| This Model is valid for Automotive grade 2 Temperature Range -40C<=Tc<=105C
| Valid for LPDDR4-4266 operation
| Part Number   VDD/VDDQ   Package   Architecture
| SCB11N8G322BF-04ZA2   1.1 +0.07/-0.04  BGA   8G bit x 32
[IBIS ver] 5.0
[File name]  usssn8g32ba2.ibs
[File Rev]  1.0
[Date]   October 8, 2023
[Source] Simulation of a silicon level SPICE model
[Notes]  IBIS Characteristics for I/O Buffer
  IBIS Model Revision History: Rev 1.0:
  2023-10-08 - IBIS model file initial creation
[Disclaimer]  The IBIS models are for modeling purpose only and are subject to change without any notice. UniIC is not
  responsible for any problems the models may cause.
[Copyright] Copyright 2023 UniIC Semiconductors Corp. All rights reserved
|   Component SCB11N8G322BF-04ZA2
[Component] SCB11N8G322BF-04ZA2
[Manufacturer] UniIC Semiconductors Corp.
[Package]
| variable   typ   min   max
R_pkg   0.750   0.698   0.832
L_pkg   1.500nH   1.330nH   1.720nH
C_pkg   0.630pF   0.579pF   0.668pF
[Pin]  signal_name   model_name   R_pin   L_pin   C_pin
A1   DNU   NC
A2   DNU   NC
A3   VSS   Gnd
A4   VDD2   Power
A5   ZQ0   NC
A8   DNU   NC
A9   VDD2   Power
A10   VSS   Gnd
A11   DNU   NC
A12   DNU   NC
AA1   DNU   NC
AA2   DQ0_B   DQ   0.835   1.840nH   0.572pF
AA3   VDDQ   Power
AA4   DQ7_B   DQ   0.804   1.770nH   0.584pF
AA5   VDDQ   Power
AA8   VDDQ   Power
AA9   DQ15_B   DQ   0.820   1.780nH   0.582pF
AA10   VDDQ   Power
AA11   DQ8_B   DQ   0.835   1.830nH   0.564pF
AA12   DNU   NC
AB1   DNU   NC
AB2   DNU   NC
AB3   VSS   Gnd
AB4   VDD2   Power
AB5   VSS   Gnd
AB8   VSS   Gnd
AB9   VDD2   Power
AB10   VSS   Gnd
AB11   DNU   NC
AB12   DNU   NC
B1   DNU   NC
B2   DQ0_A   DQ   0.825   1.680nH   0.658pF
B3   VDDQ   Power
B4   DQ7_A   DQ   0.810   1.640nH   0.579pF
B5   VDDQ   Power
B8   VDDQ   Power
B9   DQ15_A   DQ   0.819   1.720nH   0.645pF
B10   VDDQ   Power
B11   DQ8_A   DQ   0.832   1.650nH   0.595pF
B12   DNU   NC
C1   VSS   Gnd
C2   DQ1_A   DQ   0.809   1.620nH   0.658pF
C3   DMI0_A   DQ   0.816   1.600nH   0.644pF
C4   DQ6_A   DQ   0.782   1.720nH   0.645pF
C5   VSS   Gnd
C8   VSS   Gnd
C9   DQ14_A   DQ   0.776   1.550nH   0.639pF
C10   DMI1_A   DQ   0.793   1.560nH   0.644pF
C11   DQ9_A   DQ   0.809   1.640nH   0.668pF
C12   VSS   Gnd
D1   VDDQ   Power
D2   VSS   Gnd
D3   DQS0_T_A   DQS   0.752   1.480nH   0.614pF
D4   VSS   Gnd
D5   VDDQ   Power
D8   VDDQ   Power
D9   VSS   Gnd
D10   DQS1_T_A   DQS   0.750   1.460nH   0.630pF
D11   VSS   Gnd
D12   VDDQ   Power
E1   VSS   Gnd
E2   DQ2_A   DQ   0.772   1.490nH   0.579pF
E3   DQS0_C_A   DQS   0.739   1.480nH   0.613pF
E4   DQ5_A   DQ   0.698   1.360nH   0.629pF
E5   VSS   Gnd
E8   VSS   Gnd
E9   DQ13_A   DQ   0.701   1.330nH   0.647pF
E10   DQS1_C_A   DQS   0.749   1.470nH   0.622pF
E11   DQ10_A   DQ   0.786   1.530nH   0.591pF
E12   VSS   Gnd
F1   VDD1   Power
F2   DQ3_A   DQ   0.748   1.480nH   0.582pF
F3   VDDQ   Power
F4   DQ4_A   DQ   0.740   1.430nH   0.640pF
F5   VDD2   Power
F8   VDD2   Power
F9   DQ12_A   DQ   0.751   1.420nH   0.664pF
F10   VDDQ   Power
F11   DQ11_A   DQ   0.765   1.520nH   0.562pF
F12   VDD1   Power
G1   VSS   Gnd
G2   ODTCA_A   RCV_RST_N
G3   VSS   Gnd
G4   VDD1   Power
G5   VSS   Gnd
G8   VSS   Gnd
G9   VDD1   Power
G10   VSS   Gnd
G11   ZQ2   NC
G12   VSS   Gnd
H1   VDD2   Power
H2   CA0_A   CA   1.640   2.810nH   1.140pF
H3   DNU   NC
H4   CS0_A   CA   1.170   2.210nH   0.905pF
H5   VDD2   Power
H8   VDD2   Power
H9   CA2_A   CA   1.550   2.690nH   1.150pF
H10   CA3_A   CA   1.570   2.740nH   1.120pF
H11   CA4_A   CA   1.600   2.780nH   1.160pF
H12   VDD2   Power
J1   VSS   Gnd
J2   CA1_A   CA   1.670   2.970nH   1.170pF
J3   VSS   Gnd
J4   CKE0_A   RCV_CKE   1.490   2.670nH   1.000pF
J5   DNU   NC
J8   CKT_A   CLK   1.400   2.570nH   1.060pF
J9   CKC_A   CLK   1.420   2.610nH   1.070pF
J10   VSS   Gnd
J11   CA5_A   CA   1.710   2.940nH   1.200pF
J12   VSS   Gnd
K1   VDD2   Power
K2   VSS   Gnd
K3   VDD2   Power
K4   VSS   Gnd
K5   DNU   NC
K8   DNU   NC
K9   VSS   Gnd
K10   VDD2   Power
K11   VSS   Gnd
K12   VDD2   Power
N1   VDD2   Power
N2   VSS   Gnd
N3   VDD2   Power
N4   VSS   Gnd
N5   DNU   NC
N8   DNU   NC
N9   VSS   Gnd
N10   VDD2   Power
N11   VSS   Gnd
N12   VDD2   Power
P1   VSS   Gnd
P2   CA1_B   CA   1.640   4.130nH   1.160pF
P3   VSS   Gnd
P4   CKE0_B   RCV_CKE   1.370   3.590nH   1.000pF
P5   DNU   NC
P8   CKT_B   CLK   1.360   3.150nH   1.070pF
P9   CKC_B   CLK   1.420   3.190nH   1.070pF
P10   VSS   Gnd
P11   CA5_B   CA   1.610   3.550nH   1.170pF
P12   VSS   Gnd
R1   VDD2   Power
R2   CA0_B   CA   1.570   3.920nH   1.110pF
R3   NC   NC
R4   CS0_B   CA   1.240   3.090nH   0.917pF
R5   VDD2   Power
R8   VDD2   Power
R9   CA2_B   CA   1.560   3.330nH   1.170pF
R10   CA3_B   CA   1.520   3.350nH   1.140pF
R11   CA4_B   CA   1.660   3.620nH   1.200pF
R12   VDD2   Power
T1   VSS   Gnd
T2   ODTCA_B   RCV_RST_N
T3   VSS   Gnd
T4   VDD1   Power
T5   VSS   Gnd
T8   VSS   Gnd
T9   VDD1   Power
T10   VSS   Gnd
T11   RESET_N   RCV_RST_N
T12   VSS   Gnd
U1   VDD1   Power
U2   DQ3_B   DQ   0.792   1.670nH   0.563pF
U3   VDDQ   Power
U4   DQ4_B   DQ   0.775   1.610nH   0.550pF
U5   VDD2   Power
U8   VDD2   Power
U9   DQ12_B   DQ   0.731   1.520nH   0.585pF
U10   VDDQ   Power
U11   DQ11_B   DQ   0.795   1.670nH   0.572pF
U12   VDD1   Power
V1   VSS   Gnd
V2   DQ2_B   DQ   0.790   1.640nH   0.565pF
V3   DQS0_C_B   DQS   0.777   1.590nH   0.612pF
V4   DQ5_B   DQ   0.750   1.510nH   0.652pF
V5   VSS   Gnd
V8   VSS   Gnd
V9   DQ13_B   DQ   0.724   1.500nH   0.648pF
V10   DQS1_C_B   DQS   0.772   1.610nH   0.610pF
V11   DQ10_B   DQ   0.834   1.690nH   0.610pF
V12   VSS   Gnd
W1   VDDQ   Power
W2   VSS   Gnd
W3   DQS0_T_B   DQS   0.780   1.610nH   0.610pF
W4   VSS   Gnd
W5   VDDQ   Power
W8   VDDQ   Power
W9   VSS   Gnd
W10   DQS1_T_B   DQS   0.767   1.590nH   0.614pF
W11   VSS   Gnd
W12   VDDQ   Power
Y1   VSS   Gnd
Y2   DQ1_B   DQ   0.822   1.760nH   0.644pF
Y3   DMI0_B   DQ   0.812   1.630nH   0.623pF
Y4   DQ6_B   DQ   0.807   1.700nH   0.631pF
Y5   VSS   Gnd
Y8   VSS   Gnd
Y9   DQ14_B   DQ   0.841   1.720nH   0.647pF
Y10   DMI1_B   DQ   0.781   1.630nH   0.623pF
Y11   DQ9_B   DQ   0.834   1.770nH   0.633pF
Y12   VSS   Gnd
|IN   dq_in   dummy
|EN   dq_en   dummy
[Diff pin]  inv_pin  vdiff   tdelay_typ   tdelay_min   tdelay_max
D3   E3   0.160V   NA   NA   NA
D10   E10   0.160V   NA   NA   NA
J8   J9   0.160V   NA   NA   NA
V3   W3   0.160V   NA   NA   NA
V10   W10   0.160V   NA   NA   NA
P8   P9   0.160V   NA   NA   NA
[Model Selector] DQ
DQ_PU_PD_480_240_DRIVE_SOCODT240_VOH33  voh=vddq/3, 480 Ohm Pullup, 240 Ohm Pulldown,240ohm SOCODT
DQ_PU_PD_480_120_DRIVE_SOCODT240_VOH33  voh=vddq/3, 480 Ohm Pullup, 120 Ohm Pulldown,240ohm SOCODT
DQ_PU_PD_480_80_DRIVE_SOCODT240_VOH33  voh=vddq/3, 480 Ohm Pullup, 80 Ohm Pulldown,240ohm SOCODT
DQ_PU_PD_480_60_DRIVE_SOCODT240_VOH33  voh=vddq/3, 480 Ohm Pullup, 60 Ohm Pulldown,240ohm SOCODT
DQ_PU_PD_480_48_DRIVE_SOCODT240_VOH33  voh=vddq/3, 480 Ohm Pullup, 48 Ohm Pulldown,240ohm SOCODT
DQ_PU_PD_480_40_DRIVE_SOCODT240_VOH33  voh=vddq/3, 480 Ohm Pullup, 40 Ohm Pulldown,240ohm SOCODT
DQ_PU_PD_240_240_DRIVE_SOCODT120_VOH33  voh=vddq/3, 240 Ohm Pullup, 240 Ohm Pulldown,120ohm SOCODT
DQ_PU_PD_240_120_DRIVE_SOCODT120_VOH33  voh=vddq/3, 240 Ohm Pullup, 120 Ohm Pulldown,120ohm SOCODT
DQ_PU_PD_240_80_DRIVE_SOCODT120_VOH33  voh=vddq/3, 240 Ohm Pullup, 80 Ohm Pulldown,120ohm SOCODT
DQ_PU_PD_240_60_DRIVE_SOCODT120_VOH33  voh=vddq/3, 240 Ohm Pullup, 60 Ohm Pulldown,120ohm SOCODT
DQ_PU_PD_240_48_DRIVE_SOCODT120_VOH33  voh=vddq/3, 240 Ohm Pullup, 48 Ohm Pulldown,120ohm SOCODT
DQ_PU_PD_240_40_DRIVE_SOCODT120_VOH33  voh=vddq/3, 240 Ohm Pullup, 40 Ohm Pulldown,120ohm SOCODT
DQ_PU_PD_160_240_DRIVE_SOCODT80_VOH33  voh=vddq/3, 160 Ohm Pullup, 240 Ohm Pulldown,80ohm SOCODT
DQ_PU_PD_160_120_DRIVE_SOCODT80_VOH33  voh=vddq/3, 160 Ohm Pullup, 120 Ohm Pulldown,80ohm SOCODT
DQ_PU_PD_160_80_DRIVE_SOCODT80_VOH33  voh=vddq/3, 160 Ohm Pullup, 80 Ohm Pulldown,80ohm SOCODT
DQ_PU_PD_160_60_DRIVE_SOCODT80_VOH33  voh=vddq/3, 160 Ohm Pullup, 60 Ohm Pulldown,80ohm SOCODT
DQ_PU_PD_160_48_DRIVE_SOCODT80_VOH33  voh=vddq/3, 160 Ohm Pullup, 48 Ohm Pulldown,80ohm SOCODT
DQ_PU_PD_160_40_DRIVE_SOCODT80_VOH33  voh=vddq/3, 160 Ohm Pullup, 40 Ohm Pulldown,80ohm SOCODT
DQ_PU_PD_120_240_DRIVE_SOCODT60_VOH33  voh=vddq/3, 120 Ohm Pullup, 240 Ohm Pulldown,60ohm SOCODT
DQ_PU_PD_120_120_DRIVE_SOCODT60_VOH33  voh=vddq/3, 120 Ohm Pullup, 120 Ohm Pulldown,60ohm SOCODT
DQ_PU_PD_120_80_DRIVE_SOCODT60_VOH33  voh=vddq/3, 120 Ohm Pullup, 80 Ohm Pulldown,60ohm SOCODT
DQ_PU_PD_120_60_DRIVE_SOCODT60_VOH33  voh=vddq/3, 120 Ohm Pullup, 60 Ohm Pulldown,60ohm SOCODT
DQ_PU_PD_120_48_DRIVE_SOCODT60_VOH33  voh=vddq/3, 120 Ohm Pullup, 48 Ohm Pulldown,60ohm SOCODT
DQ_PU_PD_120_40_DRIVE_SOCODT60_VOH33  voh=vddq/3, 120 Ohm Pullup, 40 Ohm Pulldown,60ohm SOCODT
DQ_PU_PD_96_240_DRIVE_SOCODT48_VOH33  voh=vddq/3, 96 Ohm Pullup, 240 Ohm Pulldown,48ohm SOCODT
DQ_PU_PD_96_120_DRIVE_SOCODT48_VOH33  voh=vddq/3, 96 Ohm Pullup, 120 Ohm Pulldown,48ohm SOCODT
DQ_PU_PD_96_80_DRIVE_SOCODT48_VOH33  voh=vddq/3, 96 Ohm Pullup, 80 Ohm Pulldown,48ohm SOCODT
DQ_PU_PD_96_60_DRIVE_SOCODT48_VOH33  voh=vddq/3, 96 Ohm Pullup, 60 Ohm Pulldown,48ohm SOCODT
DQ_PU_PD_96_48_DRIVE_SOCODT48_VOH33  voh=vddq/3, 96 Ohm Pullup, 48 Ohm Pulldown,48ohm SOCODT
DQ_PU_PD_96_40_DRIVE_SOCODT48_VOH33  voh=vddq/3, 96 Ohm Pullup, 40 Ohm Pulldown,48ohm SOCODT
DQ_PU_PD_80_240_DRIVE_SOCODT40_VOH33  voh=vddq/3, 80 Ohm Pullup, 240 Ohm Pulldown,SOCODT disable OR 40ohm SOCODT
DQ_PU_PD_80_120_DRIVE_SOCODT40_VOH33  voh=vddq/3, 80 Ohm Pullup, 120 Ohm Pulldown,SOCODT disable OR 40ohm SOCODT
DQ_PU_PD_80_80_DRIVE_SOCODT40_VOH33  voh=vddq/3, 80 Ohm Pullup, 80 Ohm Pulldown,SOCODT disable OR 40ohm SOCODT
DQ_PU_PD_80_60_DRIVE_SOCODT40_VOH33  voh=vddq/3, 80 Ohm Pullup, 60 Ohm Pulldown,SOCODT disable OR 40ohm SOCODT
DQ_PU_PD_80_48_DRIVE_SOCODT40_VOH33  voh=vddq/3, 80 Ohm Pullup, 48 Ohm Pulldown,SOCODT disable OR 40ohm SOCODT
DQ_PU_PD_80_40_DRIVE_SOCODT40_VOH33  voh=vddq/3, 80 Ohm Pullup, 40 Ohm Pulldown,SOCODT disable OR 40ohm SOCODT
DQ_PU_PD_120_240_DRIVE_SOCODT80_VOH40  voh=vddq/2.5, 120 Ohm Pullup, 240 Ohm Pulldown,SOCODT disable OR 80ohm SOCODT
DQ_PU_PD_120_120_DRIVE_SOCODT80_VOH40  voh=vddq/2.5, 120 Ohm Pullup, 120 Ohm Pulldown,SOCODT disable OR 80ohm SOCODT
DQ_PU_PD_120_80_DRIVE_SOCODT80_VOH40  voh=vddq/2.5, 120 Ohm Pullup, 80 Ohm Pulldown,SOCODT disable OR 80ohm SOCODT
DQ_PU_PD_120_60_DRIVE_SOCODT80_VOH40  voh=vddq/2.5, 120 Ohm Pullup, 60 Ohm Pulldown,SOCODT disable OR 80ohm SOCODT
DQ_PU_PD_120_48_DRIVE_SOCODT80_VOH40  voh=vddq/2.5, 120 Ohm Pullup, 48 Ohm Pulldown,SOCODT disable OR 80ohm SOCODT
DQ_PU_PD_120_40_DRIVE_SOCODT80_VOH40  voh=vddq/2.5, 120 Ohm Pullup, 40 Ohm Pulldown,SOCODT disable OR 80ohm SOCODT
DQ_PU_PD_180_240_DRIVE_SOCODT120_VOH40  voh=vddq/2.5, 180 Ohm Pullup, 240 Ohm Pulldown,120ohm SOCODT
DQ_PU_PD_180_120_DRIVE_SOCODT120_VOH40  voh=vddq/2.5, 180 Ohm Pullup, 120 Ohm Pulldown,120ohm SOCODT
DQ_PU_PD_180_80_DRIVE_SOCODT120_VOH40  voh=vddq/2.5, 180 Ohm Pullup, 80 Ohm Pulldown,120ohm SOCODT
DQ_PU_PD_180_60_DRIVE_SOCODT120_VOH40  voh=vddq/2.5, 180 Ohm Pullup, 60 Ohm Pulldown,120ohm SOCODT
DQ_PU_PD_180_48_DRIVE_SOCODT120_VOH40  voh=vddq/2.5, 180 Ohm Pullup, 48 Ohm Pulldown,120ohm SOCODT
DQ_PU_PD_180_40_DRIVE_SOCODT120_VOH40  voh=vddq/2.5, 180 Ohm Pullup, 40 Ohm Pulldown,120ohm SOCODT
DQ_PU_PD_360_240_DRIVE_SOCODT240_VOH40  voh=vddq/2.5, 360 Ohm Pullup, 240 Ohm Pulldown,240ohm SOCODT
DQ_PU_PD_360_120_DRIVE_SOCODT240_VOH40  voh=vddq/2.5, 360 Ohm Pullup, 120 Ohm Pulldown,240ohm SOCODT
DQ_PU_PD_360_80_DRIVE_SOCODT240_VOH40  voh=vddq/2.5, 360 Ohm Pullup, 80 Ohm Pulldown,240ohm SOCODT
DQ_PU_PD_360_60_DRIVE_SOCODT240_VOH40  voh=vddq/2.5, 360 Ohm Pullup, 60 Ohm Pulldown,240ohm SOCODT
DQ_PU_PD_360_48_DRIVE_SOCODT240_VOH40  voh=vddq/2.5, 360 Ohm Pullup, 48 Ohm Pulldown,240ohm SOCODT
DQ_PU_PD_360_40_DRIVE_SOCODT240_VOH40  voh=vddq/2.5, 360 Ohm Pullup, 40 Ohm Pulldown,240ohm SOCODT
DQ_ODTOFF  DQ Type input, ODT off for DQ_RCV
DQ_ODT40_VOH33  voh=vddq/3, DQ Type input, ODT 40 for DQ_RCV
DQ_ODT48_VOH33  voh=vddq/3, DQ Type input, ODT 48 for DQ_RCV
DQ_ODT60_VOH33  voh=vddq/3, DQ Type input, ODT 60 for DQ_RCV
DQ_ODT80_VOH33  voh=vddq/3, DQ Type input, ODT 80 for DQ_RCV
DQ_ODT120_VOH33  voh=vddq/3, DQ Type input, ODT 120 for DQ_RCV
DQ_ODT240_VOH33  voh=vddq/3, DQ Type input, ODT 240 for DQ_RCV
DQ_ODT40_VOH40  voh=vddq/2.5, DQ Type input, ODT 40 for DQ_RCV
DQ_ODT48_VOH40  voh=vddq/2.5, DQ Type input, ODT 48 for DQ_RCV
DQ_ODT60_VOH40  voh=vddq/2.5, DQ Type input, ODT 60 for DQ_RCV
DQ_ODT80_VOH40  voh=vddq/2.5, DQ Type input, ODT 80 for DQ_RCV
DQ_ODT120_VOH40  voh=vddq/2.5, DQ Type input, ODT 120 for DQ_RCV
DQ_ODT240_VOH40  voh=vddq/2.5, DQ Type input, ODT 240 for DQ_RCV
[Model Selector] DQS
DQS_PU_PD_480_240_DRIVE_SOCODT240_VOH33  voh=vddq/3, 480 Ohm Pullup, 240 Ohm Pulldown,240ohm SOCODT
DQS_PU_PD_480_120_DRIVE_SOCODT240_VOH33  voh=vddq/3, 480 Ohm Pullup, 120 Ohm Pulldown,240ohm SOCODT
DQS_PU_PD_480_80_DRIVE_SOCODT240_VOH33  voh=vddq/3, 480 Ohm Pullup, 80 Ohm Pulldown,240ohm SOCODT
DQS_PU_PD_480_60_DRIVE_SOCODT240_VOH33  voh=vddq/3, 480 Ohm Pullup, 60 Ohm Pulldown,240ohm SOCODT
DQS_PU_PD_480_48_DRIVE_SOCODT240_VOH33  voh=vddq/3, 480 Ohm Pullup, 48 Ohm Pulldown,240ohm SOCODT
DQS_PU_PD_480_40_DRIVE_SOCODT240_VOH33  voh=vddq/3, 480 Ohm Pullup, 40 Ohm Pulldown,240ohm SOCODT
DQS_PU_PD_240_240_DRIVE_SOCODT120_VOH33  voh=vddq/3, 240 Ohm Pullup, 240 Ohm Pulldown,120ohm SOCODT
DQS_PU_PD_240_120_DRIVE_SOCODT120_VOH33  voh=vddq/3, 240 Ohm Pullup, 120 Ohm Pulldown,120ohm SOCODT
DQS_PU_PD_240_80_DRIVE_SOCODT120_VOH33  voh=vddq/3, 240 Ohm Pullup, 80 Ohm Pulldown,120ohm SOCODT
DQS_PU_PD_240_60_DRIVE_SOCODT120_VOH33  voh=vddq/3, 240 Ohm Pullup, 60 Ohm Pulldown,120ohm SOCODT
DQS_PU_PD_240_48_DRIVE_SOCODT120_VOH33  voh=vddq/3, 240 Ohm Pullup, 48 Ohm Pulldown,120ohm SOCODT
DQS_PU_PD_240_40_DRIVE_SOCODT120_VOH33  voh=vddq/3, 240 Ohm Pullup, 40 Ohm Pulldown,120ohm SOCODT
DQS_PU_PD_160_240_DRIVE_SOCODT80_VOH33  voh=vddq/3, 160 Ohm Pullup, 240 Ohm Pulldown,80ohm SOCODT
DQS_PU_PD_160_120_DRIVE_SOCODT80_VOH33  voh=vddq/3, 160 Ohm Pullup, 120 Ohm Pulldown,80ohm SOCODT
DQS_PU_PD_160_80_DRIVE_SOCODT80_VOH33  voh=vddq/3, 160 Ohm Pullup, 80 Ohm Pulldown,80ohm SOCODT
DQS_PU_PD_160_60_DRIVE_SOCODT80_VOH33  voh=vddq/3, 160 Ohm Pullup, 60 Ohm Pulldown,80ohm SOCODT
DQS_PU_PD_160_48_DRIVE_SOCODT80_VOH33  voh=vddq/3, 160 Ohm Pullup, 48 Ohm Pulldown,80ohm SOCODT
DQS_PU_PD_160_40_DRIVE_SOCODT80_VOH33  voh=vddq/3, 160 Ohm Pullup, 40 Ohm Pulldown,80ohm SOCODT
DQS_PU_PD_120_240_DRIVE_SOCODT60_VOH33  voh=vddq/3, 120 Ohm Pullup, 240 Ohm Pulldown,60ohm SOCODT
DQS_PU_PD_120_120_DRIVE_SOCODT60_VOH33  voh=vddq/3, 120 Ohm Pullup, 120 Ohm Pulldown,60ohm SOCODT
DQS_PU_PD_120_80_DRIVE_SOCODT60_VOH33  voh=vddq/3, 120 Ohm Pullup, 80 Ohm Pulldown,60ohm SOCODT
DQS_PU_PD_120_60_DRIVE_SOCODT60_VOH33  voh=vddq/3, 120 Ohm Pullup, 60 Ohm Pulldown,60ohm SOCODT
DQS_PU_PD_120_48_DRIVE_SOCODT60_VOH33  voh=vddq/3, 120 Ohm Pullup, 48 Ohm Pulldown,60ohm SOCODT
DQS_PU_PD_120_40_DRIVE_SOCODT60_VOH33  voh=vddq/3, 120 Ohm Pullup, 40 Ohm Pulldown,60ohm SOCODT
DQS_PU_PD_96_240_DRIVE_SOCODT48_VOH33  voh=vddq/3, 96 Ohm Pullup, 240 Ohm Pulldown,48ohm SOCODT
DQS_PU_PD_96_120_DRIVE_SOCODT48_VOH33  voh=vddq/3, 96 Ohm Pullup, 120 Ohm Pulldown,48ohm SOCODT
DQS_PU_PD_96_80_DRIVE_SOCODT48_VOH33  voh=vddq/3, 96 Ohm Pullup, 80 Ohm Pulldown,48ohm SOCODT
DQS_PU_PD_96_60_DRIVE_SOCODT48_VOH33  voh=vddq/3, 96 Ohm Pullup, 60 Ohm Pulldown,48ohm SOCODT
DQS_PU_PD_96_48_DRIVE_SOCODT48_VOH33  voh=vddq/3, 96 Ohm Pullup, 48 Ohm Pulldown,48ohm SOCODT
DQS_PU_PD_96_40_DRIVE_SOCODT48_VOH33  voh=vddq/3, 96 Ohm Pullup, 40 Ohm Pulldown,48ohm SOCODT
DQS_PU_PD_80_240_DRIVE_SOCODT40_VOH33  voh=vddq/3, 80 Ohm Pullup, 240 Ohm Pulldown,SOCODT disable OR 40ohm SOCODT
DQS_PU_PD_80_120_DRIVE_SOCODT40_VOH33  voh=vddq/3, 80 Ohm Pullup, 120 Ohm Pulldown,SOCODT disable OR 40ohm SOCODT
DQS_PU_PD_80_80_DRIVE_SOCODT40_VOH33  voh=vddq/3, 80 Ohm Pullup, 80 Ohm Pulldown,SOCODT disable OR 40ohm SOCODT
DQS_PU_PD_80_60_DRIVE_SOCODT40_VOH33  voh=vddq/3, 80 Ohm Pullup, 60 Ohm Pulldown,SOCODT disable OR 40ohm SOCODT
DQS_PU_PD_80_48_DRIVE_SOCODT40_VOH33  voh=vddq/3, 80 Ohm Pullup, 48 Ohm Pulldown,SOCODT disable OR 40ohm SOCODT
DQS_PU_PD_80_40_DRIVE_SOCODT40_VOH33  voh=vddq/3, 80 Ohm Pullup, 40 Ohm Pulldown,SOCODT disable OR 40ohm SOCODT
DQS_PU_PD_120_240_DRIVE_SOCODT80_VOH40  voh=vddq/2.5, 120 Ohm Pullup, 240 Ohm Pulldown,SOCODT disable OR 80ohm SOCODT
DQS_PU_PD_120_120_DRIVE_SOCODT80_VOH40  voh=vddq/2.5, 120 Ohm Pullup, 120 Ohm Pulldown,SOCODT disable OR 80ohm SOCODT
DQS_PU_PD_120_80_DRIVE_SOCODT80_VOH40  voh=vddq/2.5, 120 Ohm Pullup, 80 Ohm Pulldown,SOCODT disable OR 80ohm SOCODT
DQS_PU_PD_120_60_DRIVE_SOCODT80_VOH40  voh=vddq/2.5, 120 Ohm Pullup, 60 Ohm Pulldown,SOCODT disable OR 80ohm SOCODT
DQS_PU_PD_120_48_DRIVE_SOCODT80_VOH40  voh=vddq/2.5, 120 Ohm Pullup, 48 Ohm Pulldown,SOCODT disable OR 80ohm SOCODT
DQS_PU_PD_120_40_DRIVE_SOCODT80_VOH40  voh=vddq/2.5, 120 Ohm Pullup, 40 Ohm Pulldown,SOCODT disable OR 80ohm SOCODT
DQS_PU_PD_180_240_DRIVE_SOCODT120_VOH40  voh=vddq/2.5, 180 Ohm Pullup, 240 Ohm Pulldown,120ohm SOCODT
DQS_PU_PD_180_120_DRIVE_SOCODT120_VOH40  voh=vddq/2.5, 180 Ohm Pullup, 120 Ohm Pulldown,120ohm SOCODT
DQS_PU_PD_180_80_DRIVE_SOCODT120_VOH40  voh=vddq/2.5, 180 Ohm Pullup, 80 Ohm Pulldown,120ohm SOCODT
DQS_PU_PD_180_60_DRIVE_SOCODT120_VOH40  voh=vddq/2.5, 180 Ohm Pullup, 60 Ohm Pulldown,120ohm SOCODT
DQS_PU_PD_180_48_DRIVE_SOCODT120_VOH40  voh=vddq/2.5, 180 Ohm Pullup, 48 Ohm Pulldown,120ohm SOCODT
DQS_PU_PD_180_40_DRIVE_SOCODT120_VOH40  voh=vddq/2.5, 180 Ohm Pullup, 40 Ohm Pulldown,120ohm SOCODT
DQS_PU_PD_360_240_DRIVE_SOCODT240_VOH40  voh=vddq/2.5, 360 Ohm Pullup, 240 Ohm Pulldown,240ohm SOCODT
DQS_PU_PD_360_120_DRIVE_SOCODT240_VOH40  voh=vddq/2.5, 360 Ohm Pullup, 120 Ohm Pulldown,240ohm SOCODT
DQS_PU_PD_360_80_DRIVE_SOCODT240_VOH40  voh=vddq/2.5, 360 Ohm Pullup, 80 Ohm Pulldown,240ohm SOCODT
DQS_PU_PD_360_60_DRIVE_SOCODT240_VOH40  voh=vddq/2.5, 360 Ohm Pullup, 60 Ohm Pulldown,240ohm SOCODT
DQS_PU_PD_360_48_DRIVE_SOCODT240_VOH40  voh=vddq/2.5, 360 Ohm Pullup, 48 Ohm Pulldown,240ohm SOCODT
DQS_PU_PD_360_40_DRIVE_SOCODT240_VOH40  voh=vddq/2.5, 360 Ohm Pullup, 40 Ohm Pulldown,240ohm SOCODT
DQS_ODTOFF  DQS Type input, ODT off for DQS_RCV
DQS_ODT40_VOH33  voh=vddq/3, DQS Type input, ODT 40 for DQS_RCV
DQS_ODT48_VOH33  voh=vddq/3, DQS Type input, ODT 48 for DQS_RCV
DQS_ODT60_VOH33  voh=vddq/3, DQS Type input, ODT 60 for DQS_RCV
DQS_ODT80_VOH33  voh=vddq/3, DQS Type input, ODT 80 for DQS_RCV
DQS_ODT120_VOH33  voh=vddq/3, DQS Type input, ODT 120 for DQS_RCV
DQS_ODT240_VOH33  voh=vddq/3, DQS Type input, ODT 240 for DQS_RCV
DQS_ODT40_VOH40  voh=vddq/2.5, DQS Type input, ODT 40 for DQS_RCV
DQS_ODT48_VOH40  voh=vddq/2.5, DQS Type input, ODT 48 for DQS_RCV
DQS_ODT60_VOH40  voh=vddq/2.5, DQS Type input, ODT 60 for DQS_RCV
DQS_ODT80_VOH40  voh=vddq/2.5, DQS Type input, ODT 80 for DQS_RCV
DQS_ODT120_VOH40  voh=vddq/2.5, DQS Type input, ODT 120 for DQS_RCV
DQS_ODT240_VOH40  voh=vddq/2.5, DQS Type input, ODT 240 for DQS_RCV
[Model Selector] CA
CA_ODTOFF  CA/CS_N Type input, ODT off for CA_RCV
CA_ODT40_VOH33  voh=vddq/3, CA/CS_N Type input, 40 ohm ODT for CA_RCV
CA_ODT48_VOH33  voh=vddq/3, CA/CS_N Type input, 48 ohm ODT for CA_RCV
CA_ODT60_VOH33  voh=vddq/3, CA/CS_N Type input, 60 ohm ODT for CA_RCV
CA_ODT80_VOH33  voh=vddq/3, CA/CS_N Type input, 80 ohm ODT for CA_RCV
CA_ODT120_VOH33  voh=vddq/3, CA/CS_N Type input, 120 ohm ODT for CA_RCV
CA_ODT240_VOH33  voh=vddq/3, CA/CS_N Type input, 240 ohm ODT for CA_RCV
CA_ODT40_VOH40  voh=vddq/2.5, CA/CS_N Type input, 40 ohm ODT for CA_RCV
CA_ODT48_VOH40  voh=vddq/2.5, CA/CS_N Type input, 48 ohm ODT for CA_RCV
CA_ODT60_VOH40  voh=vddq/2.5, CA/CS_N Type input, 60 ohm ODT for CA_RCV
CA_ODT80_VOH40  voh=vddq/2.5, CA/CS_N Type input, 80 ohm ODT for CA_RCV
CA_ODT120_VOH40  voh=vddq/2.5, CA/CS_N Type input, 120 ohm ODT for CA_RCV
CA_ODT240_VOH40  voh=vddq/2.5, CA/CS_N Type input, 240 ohm ODT for CA_RCV
[Model Selector] CLK
CLK_ODTOFF  CLK Type input, ODT off for CLK_RCV
CLK_ODT40_VOH33  voh=vddq/3, CLK Type input, 40 ohm ODT for CLK_RCV
CLK_ODT48_VOH33  voh=vddq/3, CLK Type input, 48 ohm ODT for CLK_RCV
CLK_ODT60_VOH33  voh=vddq/3, CLK Type input, 60 ohm ODT for CLK_RCV
CLK_ODT80_VOH33  voh=vddq/3, CLK Type input, 80 ohm ODT for CLK_RCV
CLK_ODT120_VOH33  voh=vddq/3, CLK Type input, 120 ohm ODT for CLK_RCV
CLK_ODT240_VOH33  voh=vddq/3, CLK Type input, 240 ohm ODT for CLK_RCV
CLK_ODT40_VOH40  voh=vddq/2.5, CLK Type input, 40 ohm ODT for CLK_RCV
CLK_ODT48_VOH40  voh=vddq/2.5, CLK Type input, 48 ohm ODT for CLK_RCV
CLK_ODT60_VOH40  voh=vddq/2.5, CLK Type input, 60 ohm ODT for CLK_RCV
CLK_ODT80_VOH40  voh=vddq/2.5, CLK Type input, 80 ohm ODT for CLK_RCV
CLK_ODT120_VOH40  voh=vddq/2.5, CLK Type input, 120 ohm ODT for CLK_RCV
CLK_ODT240_VOH40  voh=vddq/2.5, CLK Type input, 240 ohm ODT for CLK_RCV
| Models and submodels in the file (186): DQ_PU_PD_480_240_DRIVE_SOCODT240_VOH33 (I/O), DQ_PU_PD_480_120_DRIVE_SOCODT240_VOH33 (I/O), DQ_PU_PD_480_80_DRIVE_SOCODT240_VOH33 (I/O), DQ_PU_PD_480_60_DRIVE_SOCODT240_VOH33 (I/O), DQ_PU_PD_480_48_DRIVE_SOCODT240_VOH33 (I/O), DQ_PU_PD_480_40_DRIVE_SOCODT240_VOH33 (I/O), DQ_PU_PD_240_240_DRIVE_SOCODT120_VOH33 (I/O), DQ_PU_PD_240_120_DRIVE_SOCODT120_VOH33 (I/O), DQ_PU_PD_240_80_DRIVE_SOCODT120_VOH33 (I/O), DQ_PU_PD_240_60_DRIVE_SOCODT120_VOH33 (I/O), DQ_PU_PD_240_48_DRIVE_SOCODT120_VOH33 (I/O), DQ_PU_PD_240_40_DRIVE_SOCODT120_VOH33 (I/O), DQ_PU_PD_160_240_DRIVE_SOCODT80_VOH33 (I/O), DQ_PU_PD_160_120_DRIVE_SOCODT80_VOH33 (I/O), DQ_PU_PD_160_80_DRIVE_SOCODT80_VOH33 (I/O), DQ_PU_PD_160_60_DRIVE_SOCODT80_VOH33 (I/O), DQ_PU_PD_160_48_DRIVE_SOCODT80_VOH33 (I/O), DQ_PU_PD_160_40_DRIVE_SOCODT80_VOH33 (I/O), DQ_PU_PD_120_240_DRIVE_SOCODT60_VOH33 (I/O), DQ_PU_PD_120_120_DRIVE_SOCODT60_VOH33 (I/O), DQ_PU_PD_120_80_DRIVE_SOCODT60_VOH33 (I/O), DQ_PU_PD_120_60_DRIVE_SOCODT60_VOH33 (I/O), DQ_PU_PD_120_48_DRIVE_SOCODT60_VOH33 (I/O), DQ_PU_PD_120_40_DRIVE_SOCODT60_VOH33 (I/O), DQ_PU_PD_96_240_DRIVE_SOCODT48_VOH33 (I/O), DQ_PU_PD_96_120_DRIVE_SOCODT48_VOH33 (I/O), DQ_PU_PD_96_80_DRIVE_SOCODT48_VOH33 (I/O), DQ_PU_PD_96_60_DRIVE_SOCODT48_VOH33 (I/O), DQ_PU_PD_96_48_DRIVE_SOCODT48_VOH33 (I/O), DQ_PU_PD_96_40_DRIVE_SOCODT48_VOH33 (I/O), DQ_PU_PD_80_240_DRIVE_SOCODT40_VOH33 (I/O), DQ_PU_PD_80_120_DRIVE_SOCODT40_VOH33 (I/O), DQ_PU_PD_80_80_DRIVE_SOCODT40_VOH33 (I/O), DQ_PU_PD_80_60_DRIVE_SOCODT40_VOH33 (I/O), DQ_PU_PD_80_48_DRIVE_SOCODT40_VOH33 (I/O), DQ_PU_PD_80_40_DRIVE_SOCODT40_VOH33 (I/O), DQ_PU_PD_360_240_DRIVE_SOCODT240_VOH40 (I/O), DQ_PU_PD_360_120_DRIVE_SOCODT240_VOH40 (I/O), DQ_PU_PD_360_80_DRIVE_SOCODT240_VOH40 (I/O), DQ_PU_PD_360_60_DRIVE_SOCODT240_VOH40 (I/O), DQ_PU_PD_360_48_DRIVE_SOCODT240_VOH40 (I/O), DQ_PU_PD_360_40_DRIVE_SOCODT240_VOH40 (I/O), DQ_PU_PD_180_240_DRIVE_SOCODT120_VOH40 (I/O), DQ_PU_PD_180_120_DRIVE_SOCODT120_VOH40 (I/O), DQ_PU_PD_180_80_DRIVE_SOCODT120_VOH40 (I/O), DQ_PU_PD_180_60_DRIVE_SOCODT120_VOH40 (I/O), DQ_PU_PD_180_48_DRIVE_SOCODT120_VOH40 (I/O), DQ_PU_PD_180_40_DRIVE_SOCODT120_VOH40 (I/O), DQ_PU_PD_120_240_DRIVE_SOCODT80_VOH40 (I/O), DQ_PU_PD_120_120_DRIVE_SOCODT80_VOH40 (I/O), DQ_PU_PD_120_80_DRIVE_SOCODT80_VOH40 (I/O), DQ_PU_PD_120_60_DRIVE_SOCODT80_VOH40 (I/O), DQ_PU_PD_120_48_DRIVE_SOCODT80_VOH40 (I/O), DQ_PU_PD_120_40_DRIVE_SOCODT80_VOH40 (I/O), DQS_PU_PD_480_240_DRIVE_SOCODT240_VOH33 (I/O), DQS_PU_PD_480_120_DRIVE_SOCODT240_VOH33 (I/O), DQS_PU_PD_480_80_DRIVE_SOCODT240_VOH33 (I/O), DQS_PU_PD_480_60_DRIVE_SOCODT240_VOH33 (I/O), DQS_PU_PD_480_48_DRIVE_SOCODT240_VOH33 (I/O), DQS_PU_PD_480_40_DRIVE_SOCODT240_VOH33 (I/O), DQS_PU_PD_240_240_DRIVE_SOCODT120_VOH33 (I/O), DQS_PU_PD_240_120_DRIVE_SOCODT120_VOH33 (I/O), DQS_PU_PD_240_80_DRIVE_SOCODT120_VOH33 (I/O), DQS_PU_PD_240_60_DRIVE_SOCODT120_VOH33 (I/O), DQS_PU_PD_240_48_DRIVE_SOCODT120_VOH33 (I/O), DQS_PU_PD_240_40_DRIVE_SOCODT120_VOH33 (I/O), DQS_PU_PD_160_240_DRIVE_SOCODT80_VOH33 (I/O), DQS_PU_PD_160_120_DRIVE_SOCODT80_VOH33 (I/O), DQS_PU_PD_160_80_DRIVE_SOCODT80_VOH33 (I/O), DQS_PU_PD_160_60_DRIVE_SOCODT80_VOH33 (I/O), DQS_PU_PD_160_48_DRIVE_SOCODT80_VOH33 (I/O), DQS_PU_PD_160_40_DRIVE_SOCODT80_VOH33 (I/O), DQS_PU_PD_120_240_DRIVE_SOCODT60_VOH33 (I/O), DQS_PU_PD_120_120_DRIVE_SOCODT60_VOH33 (I/O), DQS_PU_PD_120_80_DRIVE_SOCODT60_VOH33 (I/O), DQS_PU_PD_120_60_DRIVE_SOCODT60_VOH33 (I/O), DQS_PU_PD_120_48_DRIVE_SOCODT60_VOH33 (I/O), DQS_PU_PD_120_40_DRIVE_SOCODT60_VOH33 (I/O), DQS_PU_PD_96_240_DRIVE_SOCODT48_VOH33 (I/O), DQS_PU_PD_96_120_DRIVE_SOCODT48_VOH33 (I/O)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
